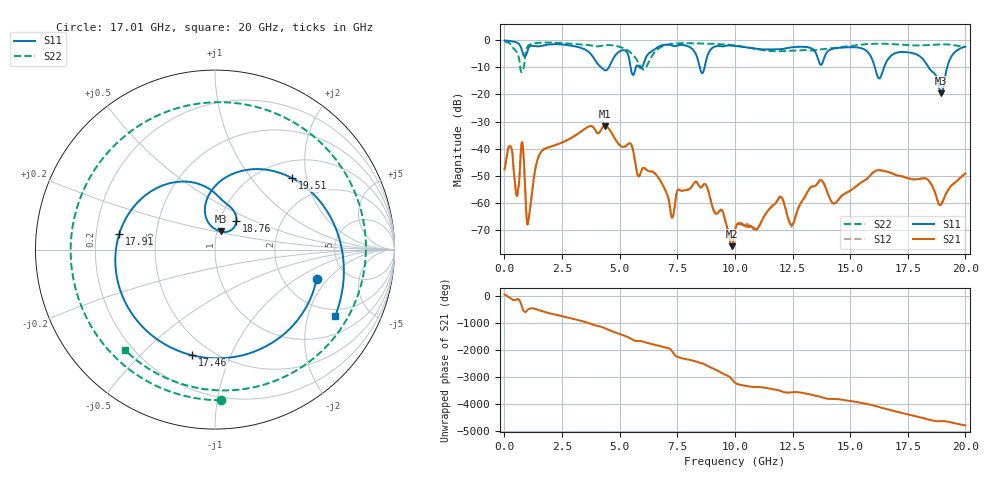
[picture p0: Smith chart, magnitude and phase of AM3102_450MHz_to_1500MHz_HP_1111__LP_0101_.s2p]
!Agilent Technologies,E8364B,MY43040894,A.07.50.67
!Agilent E8364B: A.07.50.67
!Date: Thursday, January 11, 2018 06:49:53
!Correction: S11(Full 2 Port(1,2))
!S21(Full 2 Port(1,2))
!S12(Full 2 Port(1,2))
!S22(Full 2 Port(1,2))
!S2P File: Measurements: S11, S21, S12, S22:
# Hz S  dB  R 50
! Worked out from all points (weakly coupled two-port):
!   1601 points, 10 MHz to 20 GHz, reference 50 ohm
!   highest |S21| = -31.60 dB at 4.37 GHz (marker M1); lowest = -76.0 dB at 9.868 GHz (marker M2)
!   lowest |S11| = -19.5 dB at 18.95 GHz (marker M3), VSWR 1.24, Z = 52.1 + j10.7 ohm
!   |S11| at or under -10 dB: 4.201 GHz to 4.532 GHz (330.7 MHz wide, 7.57 % of centre); 16.07 GHz to 16.47 GHz (396.6 MHz wide, 2.44 % of centre); 18.4 GHz to 19.21 GHz (809.9 MHz wide, 4.31 % of centre)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
!   |S22| runs from -11.7 to -0.4 dB; largest |S21 - S12| = 0.0014
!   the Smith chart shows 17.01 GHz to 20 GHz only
!   S11 on the Smith chart (normalised r, x): 17.01 GHz: 3.03, -1.53; 17.46 GHz: 0.39, -0.73; 17.91 GHz: 0.30, +0.07; 18.76 GHz: 1.20, +0.40; 19.51 GHz: 1.36, +1.65; 20 GHz: 1.68, -3.01
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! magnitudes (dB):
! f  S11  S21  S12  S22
! 10 MHz  -0.1  -47.7  -47.5  -0.4
! 259.9 MHz  -0.3  -39.1  -39.1  -1.3
! 547.2 MHz  -0.9  -57.4  -57.4  -4.6
! 772.1 MHz  -3.9  -37.6  -37.6  -11.4
! 1.034 GHz  -3.0  -66.8  -66.6  -2.0
! 1.572 GHz  -2.1  -41.5  -41.5  -0.9
! 3.346 GHz  -2.9  -33.6  -33.6  -1.5
! 4.37 GHz  -11.1  -31.6  -31.6  -1.8
! 6.682 GHz  -2.4  -50.8  -50.7  -3.1
! 7.281 GHz  -1.9  -65.4  -65.5  -1.3
! 8.718 GHz  -8.7  -53.2  -53.1  -1.2
! 9.868 GHz  -2.0  -76.0  -74.3  -1.8
! 10.01 GHz  -2.1  -70.5  -69.9  -1.9
! 13.34 GHz  -3.1  -54.0  -53.9  -3.8
! 16.68 GHz  -6.6  -48.7  -48.6  -1.3
! 17.01 GHz  -4.6  -49.8  -49.8  -1.5
! 17.46 GHz  -4.4  -50.8  -50.7  -1.8
! 17.91 GHz  -5.3  -51.3  -51.4  -1.9
! 18.76 GHz  -13.9  -58.5  -58.6  -1.6
! 18.95 GHz  -19.5  -60.6  -60.8  -1.5
! 19.51 GHz  -4.6  -52.7  -52.7  -1.8
! 20 GHz  -2.3  -49.2  -49.2  -2.5
